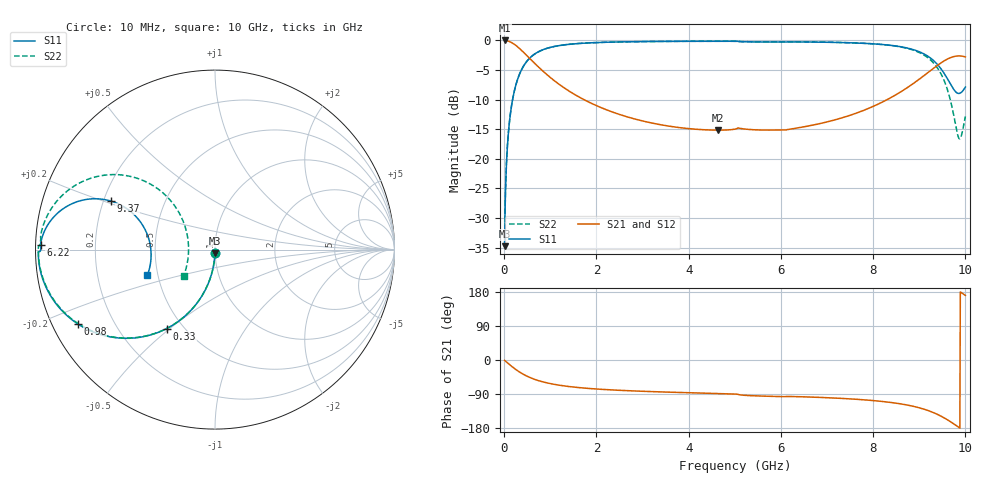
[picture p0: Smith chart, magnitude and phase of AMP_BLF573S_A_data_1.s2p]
! Created Mon Oct  5 10:30:00 2009
# ghz S ma R 50
! 2 Port Network Data from SP1.SP block
! freq  magS11  angS11  magS21  angS21  magS12  angS12  magS22  angS22
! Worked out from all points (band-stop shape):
!   1000 points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, 10 MHz to 10 GHz, reference 50 ohm
!   highest |S21| = 0.00 dB at 10 MHz (marker M1); lowest = -15.2 dB at 4.64 GHz (marker M2)
!   |S21| within 3 dB of the highest: start of sweep to 549.6 MHz; 9.648 GHz to end of sweep
!   lowest |S11| = -34.8 dB at 10 MHz (marker M3), VSWR 1.04, Z = 49.9 - j1.82 ohm
!   |S11| at or under -10 dB: start of sweep to 182.8 MHz
!   |S22| runs from -34.8 to -0.1 dB; largest |S21 - S12| = 0
!   S11 on the Smith chart (normalised r, x): 10 MHz: 1.00, -0.04; 330 MHz: 0.41, -0.49; 980 MHz: 0.07, -0.25; 6.22 GHz: 0.01, +0.01; 9.37 GHz: 0.23, +0.21; 10 GHz: 0.44, -0.15
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0.01  0.01825 -91.1  0.9998 -1.1  0.9998 -1.1  0.01825 -91.1
0.08  0.1445 -98.4  0.9895 -8.4  0.9895 -8.4  0.1445 -98.4
0.12  0.2139 -102.5  0.9768 -12.5  0.9768 -12.5  0.2139 -102.5
0.21  0.3577 -111.2  0.9338 -21.2  0.9338 -21.2  0.3577 -111.3
0.33  0.5153 -121.4  0.857 -31.5  0.857 -31.5  0.5153 -121.5
0.47  0.6497 -131.1  0.7602 -41.2  0.7602 -41.2  0.6497 -131.2
0.64  0.7574 -140.0  0.6529 -50.1  0.6529 -50.1  0.7574 -140.2
0.98  0.8694 -151.6  0.4941 -61.7  0.4941 -61.7  0.8694 -151.9
1.68  0.9462 -163.2  0.3237 -73.5  0.3237 -73.5  0.9461 -163.8
2.45  0.9706 -169.3  0.2405 -79.7  0.2405 -79.7  0.9706 -170.1
3.34  0.9807 -173.4  0.1956 -84.0  0.1956 -84.0  0.9806 -174.6
4.64  0.9846 -177.6  0.1745 -88.5  0.1745 -88.5  0.9846 -179.4
5.01  0.984 -178.9  0.1781 -89.9  0.1781 -89.9  0.9839 179.2
6.22  0.972 178.6  0.1785 -96.4  0.1785 -96.4  0.9741 175.6
6.67  0.9695 177.1  0.1917 -97.9  0.1917 -97.9  0.9712 173.7
8.34  0.9131 168.2  0.3216 -111.4  0.3216 -111.4  0.9116 161.6
8.92  0.8245 161.5  0.4463 -123.6  0.4463 -123.6  0.8148 151.5
9.37  0.6416 155.0  0.6059 -142.2  0.6059 -142.2  0.6033 138.2
9.61  0.4744 157.5  0.6963 -157.8  0.6963 -157.8  0.3847 132.2
9.85  0.3567 -178.5  0.7404 -177.1  0.7404 -177.1  0.1517 167.8
9.91  0.3636 -169.8  0.7387 177.9  0.7387 177.9  0.1552 -164.5
10  0.4039 -159.1  0.726 170.4  0.726 170.4  0.2285 -140.0
